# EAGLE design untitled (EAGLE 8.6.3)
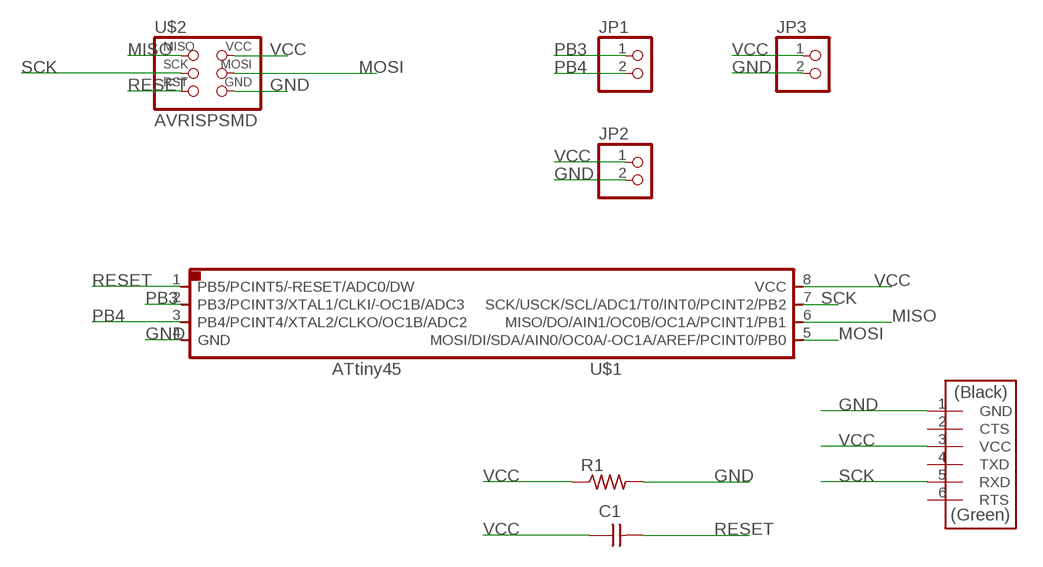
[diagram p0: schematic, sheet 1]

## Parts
C1  CAP-UNPOLARIZEDFAB  [C1206FAB]
JP1  PINHD-1X2  [1X02]
JP2  PINHD-1X2  [1X02]
JP3  PINHD-1X2  [1X02]
R1  RES-US1206FAB  [R1206FAB]
U$1  ATTINY45SI  [SOIC8]
U$2  AVRISPSMD  [2X03SMD]
U$3  FTDI-SMD-HEADER  [1X06SMD]

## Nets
GND: JP2.2 JP3.2 R1.2 U$1.4(GND) U$2.6(GND) U$3.1(GND)
MISO: U$1.6(MISO/DO/AIN1/OC0B/OC1A/PCINT1/PB1) U$2.1(MISO)
MOSI: U$1.5(MOSI/DI/SDA/AIN0/OC0A/-OC1A/AREF/PCINT0/PB0) U$2.4(MOSI)
PB3: JP1.1 U$1.2(PB3/PCINT3/XTAL1/CLKI/-OC1B/ADC3)
PB4: JP1.2 U$1.3(PB4/PCINT4/XTAL2/CLKO/OC1B/ADC2)
RESET: C1.2 U$1.1(PB5/PCINT5/-RESET/ADC0/DW) U$2.5(RST)
SCK: U$1.7(SCK/USCK/SCL/ADC1/T0/INT0/PCINT2/PB2) U$2.3(SCK) U$3.5(RXD)
VCC: C1.1 JP2.1 JP3.1 R1.1 U$1.8(VCC) U$2.2(VCC) U$3.3(VCC)
Unconnected: U$3.2(CTS) U$3.4(TXD) U$3.6(RTS)

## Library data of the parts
C1 = 001_fab:CAP-UNPOLARIZED
JP1-JP3 = pinhead:PINHD-1X2: PIN HEADER
R1 = 001_fab:RES-US: Resistor (US Symbol)
U$1 = 001_fab:ATTINY45
U$2 = 001_fab:AVRISP
U$3 = 001_fab:FTDI-SMD-HEADER

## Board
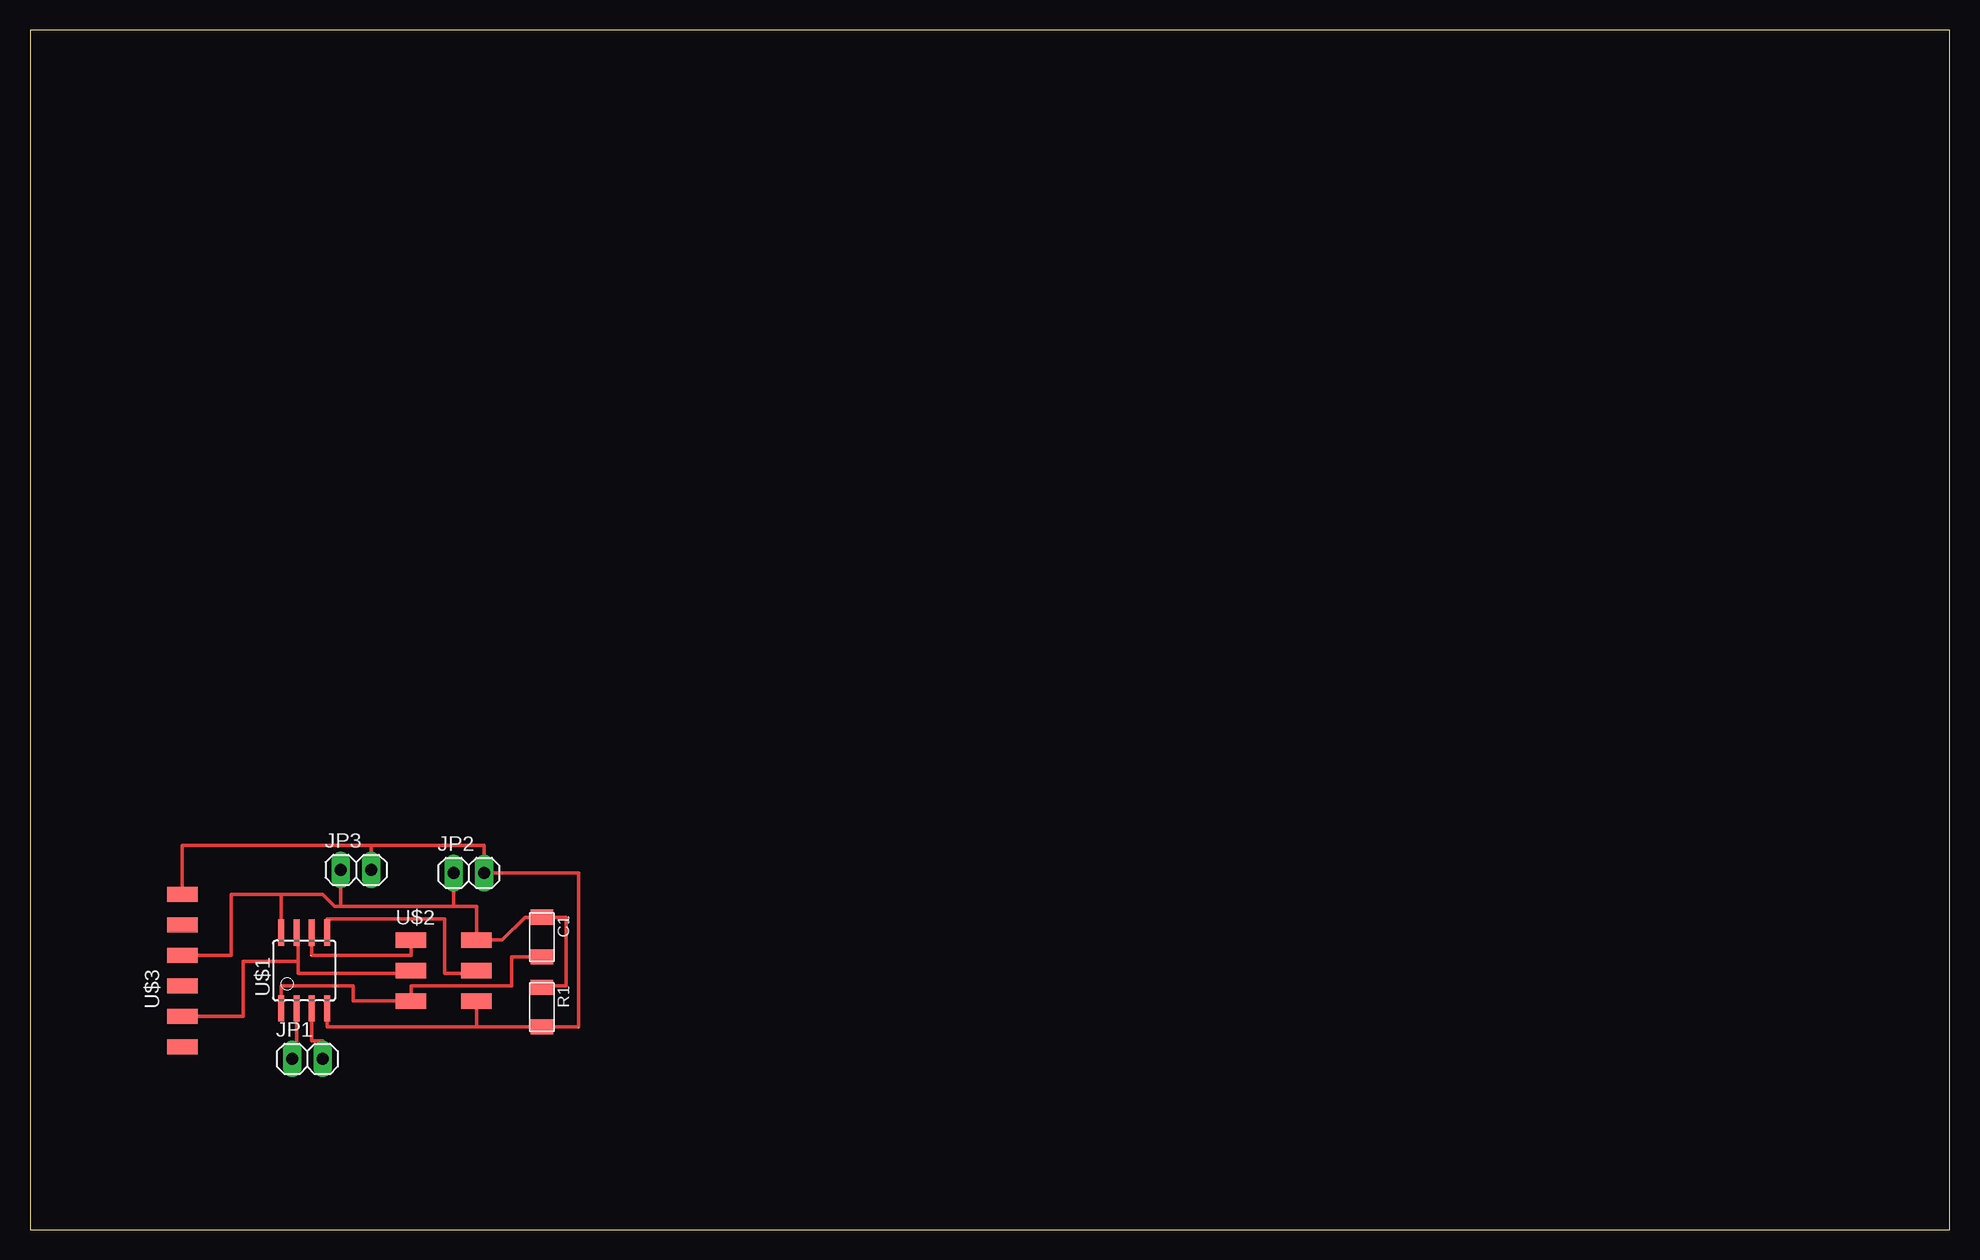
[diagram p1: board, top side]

Size 160 x 100 mm. Coordinates in mm from the lower left corner, seen from the top.
Outline: 0,0 160,0 160,100 0,100 0,0
Copper layers (1*16): Top 0.035mm / dielectric 1.5mm / Bottom 0.035mm
Design rules "default": minimum track width 6mil, minimum drill 0.35mm, track to track 6mil, track to pad 6mil, pad to pad 6mil, via to via 6mil, smd to smd 6mil, copper to edge 40mil, drill to drill 6mil, minimum pad ring 10mil, minimum via ring 8mil, stop-mask expansion 4mil, vias tented up to drill 0mil, thermal gap 10mil

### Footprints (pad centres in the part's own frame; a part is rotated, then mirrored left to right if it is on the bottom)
C1206FAB = smd 1.27 x 1.905: 1 -1.651,0; 2 1.651,0
1X02 = drill 1.016 long: 1 -1.27,0; 2 1.27,0
R1206FAB = smd 1.27 x 1.905: 1 -1.651,0; 2 1.651,0
SOIC8 = smd 0.5 x 2.2: 1 -1.905,-3.154; 2 -0.645,-3.154; 3 0.625,-3.154; 4 1.895,-3.154; 5 1.905,3.154; 6 0.635,3.154; 7 -0.635,3.154; 8 -1.905,3.154
2X03SMD = smd 2.54 x 1.27: 1 -2.54,2.54; 2 2.92,2.54; 3 -2.54,0; 4 2.92,0; 5 -2.54,-2.54; 6 2.92,-2.54
1X06SMD = smd 2.54 x 1.27: 1 0,6.35; 2 0,3.81; 3 0,1.27; 4 0,-1.27; 5 0,-3.81; 6 0,-6.35

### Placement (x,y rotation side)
C1  42.67,24.38 270 top
JP1  23.11,14.22 0 top
JP2  36.58,29.72 0 top
JP3  27.18,29.97 0 top
R1  42.67,18.54 270 top
U$1  22.86,21.59 0 top
U$2  34.29,21.59 0 top
U$3  12.7,21.59 0 top

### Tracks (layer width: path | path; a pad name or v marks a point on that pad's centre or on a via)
GND  (1 unrouted)
  Top 0.305: U$3.1 12.7,32 28.45,32 | 28.45,32 37.85,32 JP2.2 45.72,29.72 45.72,16.89 R1.2 37.21,16.89 | JP3.2 28.45,32 | U$1.4 24.75,16.89 37.21,16.89 | U$2.6 37.21,16.89
MISO  (1 unrouted)
  Top 0.305: U$2.1 31.75,22.86 23.5,22.86 U$1.6
MOSI
  Top 0.305: U$1.5 24.77,25.91 34.54,25.91 34.54,21.34 37.21,21.34 U$2.4
PB3
  Top 0.305: JP1.1 22.21,14.22 U$1.2
PB4
  Top 0.305: JP1.2 24.38,15.75 23.48,15.75 U$1.3
RESET
  Top 0.305: C1.2 40.13,22.73 40.13,20.32 31.75,20.32 U$2.5 26.92,19.05 26.92,20.32 20.95,20.32 U$1.1
SCK
  Top 0.305: U$3.5 17.78,17.78 17.78,22.35 22.35,22.35 | 22.35,22.35 22.35,24.74 U$1.7 | 22.35,22.35 22.35,21.34 31.75,21.34 U$2.3
VCC
  Top 0.305: U$3.3 16.76,22.86 16.76,27.94 20.95,27.94 | 20.95,27.94 24.38,27.94 25.4,26.92 25.91,26.92 | 25.91,26.92 35.31,26.92 | 35.31,26.92 37.21,26.92 U$2.2 39.37,24.13 41.27,26.04 C1.1 44.7,26.04 44.7,20.32 42.67,20.32 R1.1 | JP2.1 35.31,26.92 | JP3.1 25.91,26.92 | U$1.8 20.95,27.94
